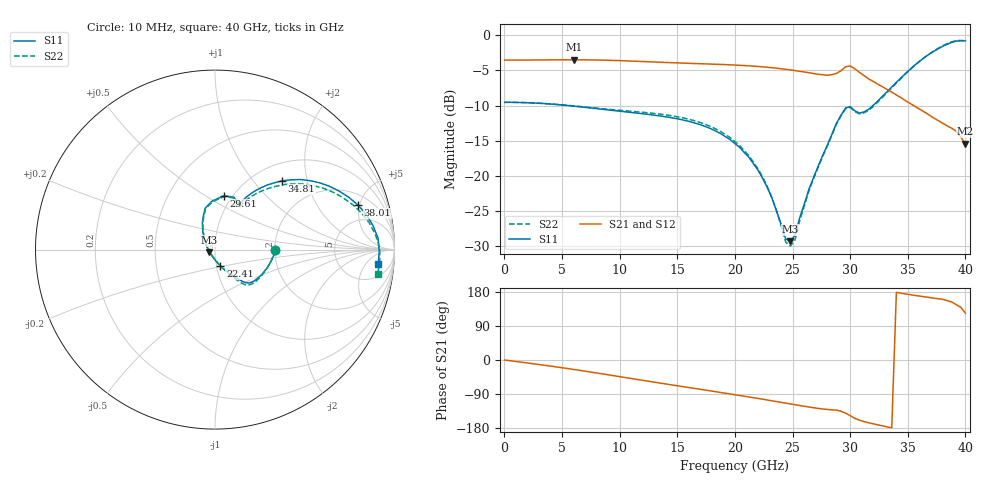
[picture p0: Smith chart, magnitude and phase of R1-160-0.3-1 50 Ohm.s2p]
!version-1
!date-09.2020
# MHz S RI R 50
!Freq ReS11 ImS11 ReS21 ImS21 ReS12 ImS12 ReS22 ImS22
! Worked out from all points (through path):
!   101 points, 10 MHz to 40 GHz, reference 50 ohm
!   highest |S21| = -3.48 dB at 6.01 GHz (marker M1); lowest = -15.5 dB at 40 GHz (marker M2)
!   group delay of S21, straight-line fit = 15.1 ps
!   lowest |S11| = -29.3 dB at 24.81 GHz (marker M3), VSWR 1.07, Z = 47 - j1.4 ohm
!   |S11| at or under -10 dB: 5.488 GHz to 31.98 GHz (26.49 GHz wide, 141 % of centre)
!   |S22| runs from -30.0 to -0.7 dB; largest |S21 - S12| = 0
!   S11 on the Smith chart (normalised r, x): 10 MHz: 2.00, -0.00; 22.41 GHz: 1.05, -0.19; 29.61 GHz: 0.91, +0.60; 34.81 GHz: 1.32, +1.42; 38.01 GHz: 2.94, +4.81; 40 GHz: 11, -11
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10  0.3334 -6.86e-05  0.6666 -0.000473  0.6666 -0.000473  0.3334 -5.83e-05
6010  0.3022 -0.0819  0.6075 -0.2825  0.6075 -0.2825  0.304 -0.0804
6810  0.2921 -0.098  0.5877 -0.3207  0.5877 -0.3207  0.2942 -0.0974
13610  0.1909 -0.185  0.3078 -0.5645  0.3078 -0.5645  0.1912 -0.1963
17210  0.1469 -0.1738  0.1262 -0.6144  0.1262 -0.6144  0.1462 -0.1851
20010  0.0929 -0.1412  -0.0183 -0.6141  -0.0183 -0.6141  0.093 -0.1475
22410  0.0305 -0.0905  -0.1402 -0.58  -0.1402 -0.58  0.0321 -0.0921
23210  0.00927 -0.0686  -0.1787 -0.5604  -0.1787 -0.5604  0.0114 -0.0691
24410  -0.0203 -0.029  -0.2321 -0.524  -0.2321 -0.524  -0.0177 -0.0286
24810  -0.0307 -0.0149  -0.2478 -0.5101  -0.2478 -0.5101  -0.028 -0.0143
25210  -0.0375 0.00118  -0.2636 -0.4956  -0.2636 -0.4956  -0.0348 0.00177
26810  -0.0625 0.0735  -0.3136 -0.4339  -0.3136 -0.4339  -0.0598 0.0734
28810  -0.0552 0.2299  -0.3601 -0.3961  -0.3601 -0.3961  -0.0526 0.2275
29610  0.0495 0.3  -0.4603 -0.3816  -0.4603 -0.3816  0.0528 0.2963
30410  0.1272 0.2602  -0.518 -0.2534  -0.518 -0.2534  0.1312 0.2544
31210  0.1368 0.2502  -0.4919 -0.1553  -0.4919 -0.1553  0.1417 0.2424
33610  0.2562 0.3442  -0.3944 -0.00678  -0.3944 -0.00678  0.2663 0.3289
34810  0.3744 0.3833  -0.3406 0.0342  -0.3406 0.0342  0.3885 0.3628
36410  0.5825 0.3723  -0.2778 0.0649  -0.2778 0.0649  0.6022 0.3423
38010  0.7962 0.2489  -0.2232 0.0802  -0.2232 0.0802  0.8161 0.2045
39210  0.9088 0.0625  -0.1719 0.1161  -0.1719 0.1161  0.9182 0.00756
40000  0.9097 -0.0828  -0.0932 0.1407  -0.0932 0.1407  0.9064 -0.1372
